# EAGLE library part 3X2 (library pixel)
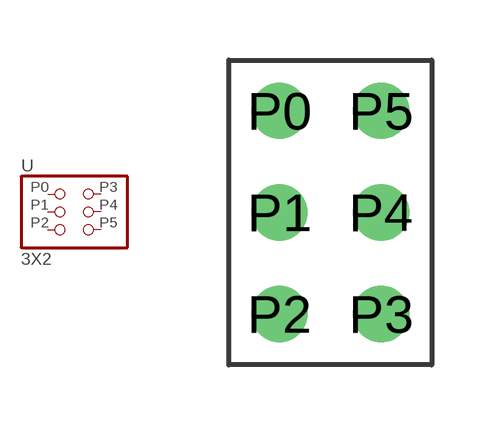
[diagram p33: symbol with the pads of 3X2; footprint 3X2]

Designator prefix -

## 3X2  [3X2]
P0  P0  pas
P1  P1  pas
P2  P2  pas
P3  P3  pas
P4  P4  pas
P5  P5  pas

## Footprint 3X2 (pad centres in mm)
drill 0.9 pad 1.27: P0 -1.27,2.54; P1 -1.27,0; P2 -1.27,-2.54; P3 1.27,-2.54; P4 1.27,0; P5 1.27,2.54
